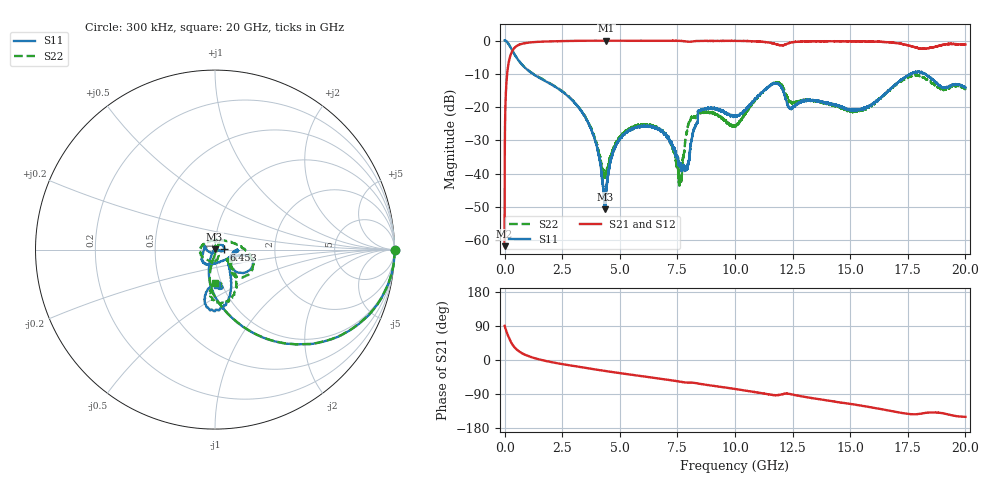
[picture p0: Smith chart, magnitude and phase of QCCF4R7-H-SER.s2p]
!QCCF4R7
!Johanson Technology Inc.
!www.johansontechnology.com
!Test Board Conditions:
!Substrate Type  RO4350B
!Substrate Thickness  10 mil
!Substrate Dk  3.66
!TL Type: GCPW
!TL Trace Width  21 mil
!TL Gap  20 mil
!Electrode orientation  Horizontal
!DUT TOPOLOGY	SERIES
!Mounting Pad LxW  16x21 mil
# MHz S  dB  R 50
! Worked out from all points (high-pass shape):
!   20001 points, 300 kHz to 20 GHz, reference 50 ohm
!   highest |S21| = -0.02 dB at 4.409 GHz (marker M1); lowest = -61.7 dB at 300 kHz (marker M2)
!   |S21| within 3 dB of the highest: 341.2 MHz to end of sweep
!   lowest |S11| = -50.7 dB at 4.347 GHz (marker M3), VSWR 1.01, Z = 49.8 + j0.169 ohm
!   |S11| at or under -10 dB: 1.23 GHz to 17.61 GHz (16.38 GHz wide, 174 % of centre); 17.62313 GHz to 17.63793 GHz (14.8 MHz wide, 0.084 % of centre); 18.24 GHz to end of sweep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
!   |S22| runs from -43.8 to 0.0 dB; largest |S21 - S12| = 0.021
!   S11 on the Smith chart (normalised r, x): 300 kHz: open; 6.453 GHz: 1.11, +0.00; 20 GHz: 0.95, -0.39
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0.3  0.04 -0.1  -61.73 90.1  -61.49 89.7  0.03 -0.1
116.298  -0.49 -20.6  -9.61 69.2  -9.64 69.3  -0.50 -20.7
351.295  -3.20 -49.7  -2.91 39.7  -2.89 39.9  -3.21 -49.8
1088.284  -9.31 -80.8  -0.58 9.0  -0.57 8.9  -9.25 -80.6
3334.25  -21.23 -111.2  -0.06 -19.3  -0.06 -19.3  -21.13 -103.2
3947.241  -30.41 -124.1  -0.03 -25.1  -0.04 -25.1  -30.04 -93.8
4347.235  -50.65 144.7  -0.02 -28.8  -0.03 -28.8  -41.03 -16.5
4409.234  -45.25 99.4  -0.02 -29.4  -0.03 -29.4  -39.59 -1.1
4964.226  -29.93 50.6  -0.04 -34.2  -0.04 -34.3  -29.27 54.6
6453.203  -25.85 0.7  -0.05 -46.9  -0.06 -46.9  -25.51 84.6
6667.2  -26.80 -4.0  -0.05 -48.7  -0.06 -48.7  -26.39 86.0
7613.186  -37.19 2.2  -0.10 -57.1  -0.10 -57.1  -42.50 23.9
7912.181  -38.29 -43.5  -0.30 -59.6  -0.31 -59.5  -27.54 -63.3
8148.178  -28.64 -163.8  -0.29 -59.8  -0.29 -59.7  -23.06 -95.8
8488.173  -21.03 -144.7  -0.11 -63.0  -0.14 -63.0  -21.65 -153.0
10000.15  -22.66 -69.5  -0.08 -76.6  -0.10 -76.3  -25.65 89.0
11719.12  -12.92 -22.1  -0.98 -92.7  -0.98 -93.1  -12.73 -24.2
12393.11  -20.34 -25.0  -0.65 -89.8  -0.66 -89.8  -18.35 -44.5
13334.1  -18.05 -2.0  -0.23 -100.3  -0.26 -100.4  -17.99 -26.0
16667.05  -15.01 -60.4  -0.52 -133.3  -0.49 -133.9  -14.93 -50.6
17910.03  -9.46 -89.3  -2.21 -142.8  -2.29 -142.9  -10.44 -84.1
20000  -14.12 -86.2  -1.17 -150.1  -1.03 -149.3  -14.51 -90.3
